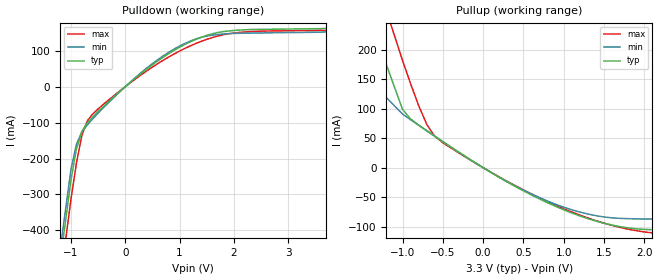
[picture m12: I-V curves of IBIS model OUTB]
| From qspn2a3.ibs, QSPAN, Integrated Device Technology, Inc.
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|   Model OUTB
[Model]   OUTB
Model_type   Output
Polarity   Non-Inverting
C_comp   5.00pF   5.00pF   5.00pF
[Voltage Range]   3.3000V   3.0000V   3.5000V
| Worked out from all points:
|   slope of the pulldown table from 0 to 0.495 V, typ, clamps not added: 8.19 ohm
|   slope of the pullup table from 0 to 0.495 V, typ, clamps not added: 12.7 ohm
[Pulldown]
| voltage   I(typ)   I(min)   I(max)
-3.3V     -3.036A    -3.001A    -3.093A
-1.5V     -828mA     -790.5mA   -888.2mA
-1V       -258.8mA   -229mA     -312.4mA
-900mV    -172.7mA   -160.1mA   -212.7mA
-800mV    -124.4mA   -125.9mA   -135.4mA
-700mV    -100.9mA   -106.5mA   -95.31mA
-500mV    -69.01mA   -73.28mA   -61.83mA
200mV     25.72mA    27.27mA    22.91mA
1V        109.7mA    113mA      99.07mA
1.4V      137.5mA    137.3mA    126.1mA
2V        156.3mA    148.1mA    149.3mA
3.7V      162mA      152.5mA    156.5mA
[Pullup]
| voltage   I(typ)   I(min)   I(max)
-3.3V     1.071A     928.4mA    1.178A
-1.7V     372.7mA    236.2mA    478mA
-1.5V     287.7mA    160.6mA    391.8mA
-1V       98.94mA    90.94mA    181.9mA
-800mV    72.32mA    71.85mA    105.3mA
-700mV    62.91mA    62.44mA    73.61mA
-600mV    53.56mA    53.13mA    53.21mA
-500mV    44.32mA    43.94mA    42.33mA
300mV     -24.37mA   -23.78mA   -23.28mA
900mV     -65.6mA    -62.02mA   -63.68mA
1.5V      -94.12mA   -83.54mA   -94.04mA
2.1V      -105.1mA   -87.03mA   -110.5mA
[Ramp]
| variable   typ   min   max
dV/dt_r   1.5666/0.7711n   1.4154/0.7899n   1.6446/0.8593n
dV/dt_f   1.6987/0.8630n   1.5596/0.6387n   1.7611/1.1934n
R_load = 50.0000
| End [Model] OUTB
| End [Component] QSpan
